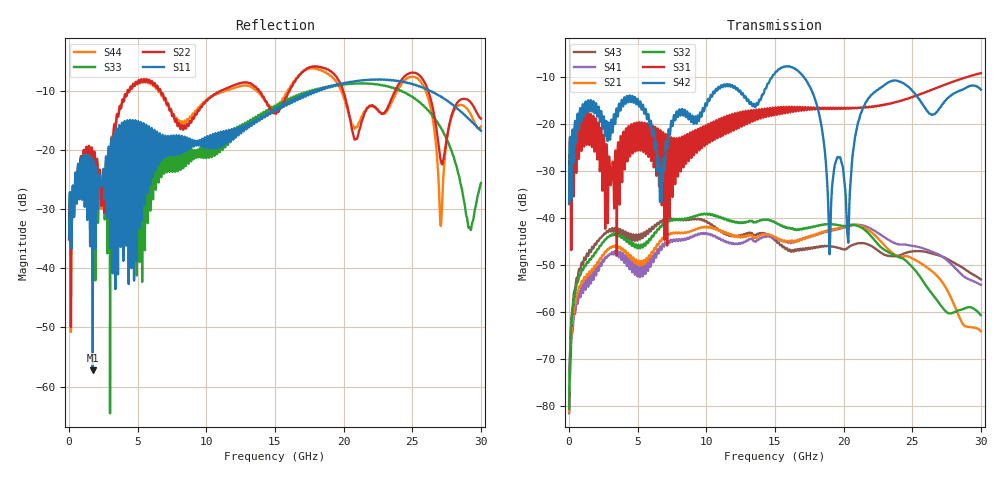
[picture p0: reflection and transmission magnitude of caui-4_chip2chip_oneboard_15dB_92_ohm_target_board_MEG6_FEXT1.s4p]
! Touchstone file from project caui-4_chip2chip_oneboard
! Exported from Circuit Design 8.0.0
! Variables:
!  $ModelNames_Index = 0
!  $ModelNames_Index1 = 0
!  $ModelNames_Index2 = 0
!  $ModelNames_Index3 = 0
!  $ModelNames_Index4 = 0
!  $ModelNames_Index5 = 0
!  Lbo = 0.5in
!  Lmain = 16in
!  lcap = 0.25in
# GHZ S MA R 50.000000
! Modal data exported
! Port[1] = Port1
! Port[2] = Port2
! Port[3] = Port3
! Port[4] = Port4
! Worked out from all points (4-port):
!   3000 points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, 10 MHz to 30 GHz, reference 50 ohm
!   strongest paths, dB at 10 MHz, 7.51 GHz, 15.01 GHz, 22.51 GHz, 30 GHz:
!     S42: -36.9, -20.0, -9.0, -12.6, -12.6
!     S31: -37.0, -29.0, -16.7, -16.0, -9.1
!     S32: -80.6, -40.4, -41.0, -45.5, -60.6
!     S21: -81.2, -43.3, -44.1, -44.3, -64.1
!     S41: -81.5, -45.0, -44.3, -43.1, -54.2
!     S43: -80.1, -40.2, -44.7, -46.9, -53.0
!   lowest |S11| = -57.2 dB at 1.73 GHz (marker M1), VSWR 1.00, Z = 50 + j0.133 ohm
!   |S11| at or under -10 dB: start of sweep to 17.89 GHz; 17.96 GHz to 18.07 GHz (111.9 MHz wide, 0.622 % of centre); 26.27 GHz to end of sweep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
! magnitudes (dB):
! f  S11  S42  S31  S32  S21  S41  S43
! 10 MHz  -34.9  -36.9  -37.0  -80.6  -81.2  -81.5  -80.1
! 1.73 GHz  -57.2  -15.9  -19.5  -48.1  -50.9  -51.9  -46.2
! 6.71 GHz  -21.8  -29.5  -24.3  -41.8  -44.9  -46.6  -40.8
! 16.33 GHz  -11.4  -8.0  -17.3  -42.3  -45.0  -45.1  -47.0
! 20.3 GHz  -8.6  -43.9  -16.6  -41.5  -41.6  -41.8  -46.3
! 22.09 GHz  -8.2  -13.6  -16.1  -44.1  -43.1  -42.4  -46.0
! 30 GHz  -16.8  -12.6  -9.1  -60.6  -64.1  -54.2  -53.0
